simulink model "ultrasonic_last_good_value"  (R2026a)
settings: Solver=FixedStepAuto  StopTime=inf  EnableMultiTasking=on
libraries: arduinosensorlib x1

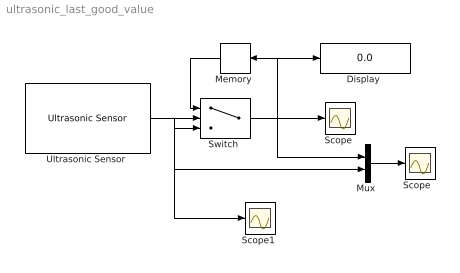
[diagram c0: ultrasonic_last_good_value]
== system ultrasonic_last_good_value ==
  "Display " : Display
  "Memory " : Memory
  "Mux " : Mux  Inputs=2
  "Scope " : Scope
  "Scope  " : Scope
  "Scope1 " : Scope
  "Switch " : Switch  Criteria=u2 > Threshold  Threshold=0.2
  "Ultrasonic Sensor " : arduinosensorlib/Ultrasonic Sensor  NumSignalPins=2  TrigPin=4  EchoPin=5  SignalPin=3  SampleTime_=0.01  blockPlatform=ARDUINO
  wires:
  "Ultrasonic Sensor "/1 -> "Switch "/3, "Scope1 "/1, "Mux "/2, "Switch "/2
  "Memory "/1 -> "Switch "/1
  "Mux "/1 -> "Scope  "/1
  "Switch "/1 -> "Memory "/1, "Display "/1, "Mux "/1, "Scope "/1
